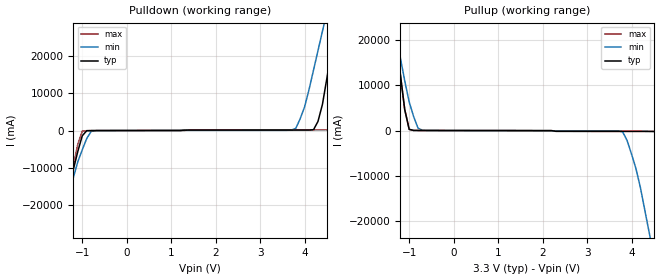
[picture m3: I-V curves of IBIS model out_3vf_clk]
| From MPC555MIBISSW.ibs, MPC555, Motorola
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| OUTPUT_3vf_clk(clk pad with 90pf load - full strength)
[Model]   out_3vf_clk
Model_type   Output
Polarity   Non-Inverting
|   typ   min   max
C_comp   5.3910e-13   4.7930e-13   6.1770e-13
| CAP models
| typical : model= typ
| maximum : model= wcs
| minimum : model= bcs
[Voltage range]   3.3v   3.0v   3.6v
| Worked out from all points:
|   slope of the pulldown table from 0 to 0.495 V, typ, clamps not added: 72.6 ohm
|   slope of the pullup table from 0 to 0.495 V, typ, clamps not added: 66 ohm
|  typical: model = typ,  temp = 25,  vdd = 3.3
|  maximum: model = bcs,  temp = -40, vdd = 3.6
|  minimum: model = wcs,  temp = 150, vdd = 3.0
[Pulldown]
|  Voltage   I(typ)   I(min)   I(max)
-3.3V     -173.6A    -120.2A    -224.6A
-1.5V     -31.57A    -27.78A    -35.88A
-1.4V     -24.48A    -22.71A    -26.9A
-1.2V     -10.44A    -12.6A     -9.348A
-1V       -1.4A      -5.157A    -139.4mA
-700mV    -12.3mA    -25.32mA   -20.14mA
3.8V      117.7mA    570.5mA    196.3mA
4.3V      2.448A     21.5A      199.2mA
4.6V      21.38A     37.15A     456.3mA
4.7V      28.72A     42.36A     4.859A
5V        50.73A     58.02A     31.4A
6.6V      209.5A     170.9A     227.7A
[Pullup]
-3.3V     267.4A     148.5A     267.4A
-1.4V     31.2A      26.66A     31.2A
-1.3V     21.88A     21.45A     21.88A
-1.1V     4.66A      11.04A     4.66A
-1V       265.4mA    6.358A     265.4mA
-700mV    12.48mA    54.68mA    12.48mA
3.8V      -184.9mA   -286mA     -184.9mA
4.1V      -186.6mA   -8.444A    -186.6mA
4.4V      -193.8mA   -22.77A    -193.8mA
4.6V      -307.9mA   -32.9A     -307.9mA
5V        -27.09A    -53.17A    -27.09A
6.6V      -189.3A    -140.2A    -189.3A
| RAMP models
| typical dv/dt : model=typ, temp=25
| maximum dv/dt : model=bcs, temp=-40
| minimum dv/dt : model=wcs, temp=150
|   typ   min   max
[Ramp]
dV/dt_r 1.4161/2.64168E-10  1.01623/1.1088e-08   1.92219/2.0188E-10
dV/dt_f 1.70008/2.4756e-10  1.28863/5.53499e-10   1.9939/1.38106e-10
